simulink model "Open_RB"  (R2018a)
settings: Solver=ode45  StartTime=0.0  StopTime=30  RelTol=1e-3  EnableMultiTasking=on
InitFcn:
  | init
undefined symbols (not defined in the file or in its folder): Av, Bv, Cv, Dv, Kmix, Kpr, Kq

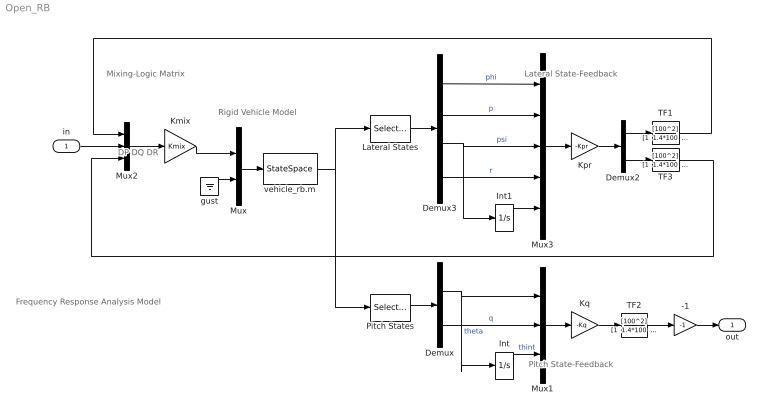
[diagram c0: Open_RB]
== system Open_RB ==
  note: Frequency Response Analysis Model
  note: Rigid Vehicle Model
  note: Pitch State-Feedback
  note: Lateral State-Feedback
  note: Mixing-Logic Matrix
  note: DP DQ DR
  in : Inport
  -1 : Gain  Gain=-1
  Demux : Demux  Outputs=2
  Demux2 : Demux  Outputs=2
  Demux3 : Demux
  Int : Integrator
  Int1 : Integrator
  Kmix : Gain  Gain=Kmix  Multiplication=Matrix(K*u)
  Kpr : Gain  Gain=-Kpr  Multiplication=Matrix(K*u)
  Kq : Gain  Gain=-Kq  Multiplication=Matrix(K*u)
  Lateral States : Selector  InputPortWidth=14  IndexOptions=Index vector (dialog)  Indices=[1,2, 5,6]  OutputSizes=1
  Mux : Mux  Inputs=[6,1]
  Mux1 : Mux  Inputs=3
  Mux2 : Mux  Inputs=3
  Mux3 : Mux  Inputs=5
  Pitch States : Selector  InputPortWidth=14  IndexOptions=Index vector (dialog)  Indices=[3, 4]  OutputSizes=1
  TF1 : TransferFcn  Numerator=[100^2]  Denominator="[1  1.4*100  100^2]"
  TF2 : TransferFcn  Numerator=[100^2]  Denominator="[1  1.4*100  100^2]"
  TF3 : TransferFcn  Numerator=[100^2]  Denominator="[1  1.4*100  100^2]"
  gust : Ground
  vehicle_rb.m : StateSpace  A=Av  B=Bv  C=Cv  D=Dv  InitialCondition=0
  out : Outport
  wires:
  Mux/1 -> vehicle_rb.m/1
  Kmix/1 -> Mux/1
  gust/1 -> Mux/2
  vehicle_rb.m/1 -> Lateral States/1, Pitch States/1
  Demux/2 -> Mux1/2  "q"
  Pitch States/1 -> Demux/1
  Mux1/1 -> Kq/1
  Demux/1 -> Int/1, Mux1/1  "theta"
  Kq/1 -> TF2/1
  Demux3/2 -> Mux3/2  "p"
  Demux3/4 -> Mux3/4  "r"
  Demux3/3 -> Mux3/3, Int1/1  "psi"
  Kpr/1 -> Demux2/1
  Demux2/1 -> TF1/1
  Demux2/2 -> TF3/1
  Demux3/1 -> Mux3/1  "phi"
  Lateral States/1 -> Demux3/1
  Mux3/1 -> Kpr/1
  Int1/1 -> Mux3/5
  Mux2/1 -> Kmix/1
  -1/1 -> out/1
  TF3/1 -> Mux2/3
  TF2/1 -> -1/1
  in/1 -> Mux2/2
  TF1/1 -> Mux2/1
  Int/1 -> Mux1/3  "thint"
